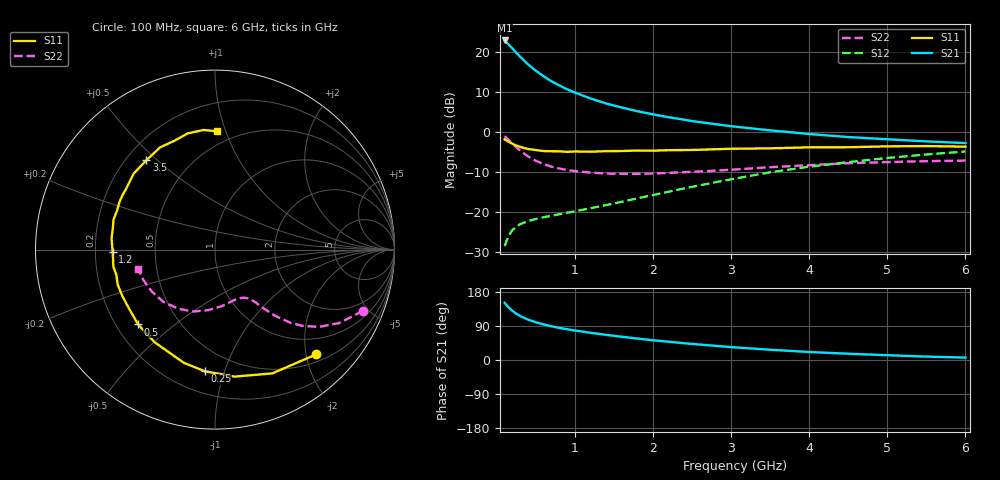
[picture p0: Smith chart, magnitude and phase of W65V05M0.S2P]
! SIEMENS Small Signal Semiconductors
! BFR193W
! Si NPN RF Bipolar Junction Transistor in SOT323
! VCE = 5 V  IC = 5 mA
! Common Emitter S-Parameters:  September  1992
# GHz  S  MA  R  50
!  f  S11  S21  S12  S22
! GHz  MAG  ANG  MAG  ANG  MAG  ANG  MAG  ANG
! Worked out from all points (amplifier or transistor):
!   28 points, 100 MHz to 6 GHz, reference 50 ohm
!   highest |S21| = 22.9 dB at 100 MHz (marker M1)
!   |S21| within 3 dB of that: start of sweep to 246.8 MHz
!   unconditionally stable (mu >= 1): 1.199 GHz to 2.565 GHz
!   at 300 MHz: K = 0.36, MSG = 20.9 dB, |S12| = -23.0 dB
!   at 1.5 GHz: K = 1.06, MAG = 10.7 dB, |S12| = -17.8 dB
!   at 6 GHz: K = 0.90, MSG = 1.0 dB, |S12| = -4.8 dB
!   lowest NFmin = 1.20 dB at 450 MHz
!   S11 on the Smith chart (normalised r, x): 100 MHz: 0.64, -2.19; 250 MHz: 0.34, -0.86; 500 MHz: 0.29, -0.38; 1.2 GHz: 0.27, -0.01; 3.5 GHz: 0.28, +0.46; 6 GHz: 0.40, +0.94
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0.1  0.811 -46.1  13.92 150.8  0.0378 67.1  0.8923 -22.5
0.15  0.76 -65.2  12.46 139.1  0.0508 58.7  0.8041 -30.6
0.2  0.7159 -81.3  11.05 129.7  0.0598 52.8  0.7211 -36.7
0.25  0.6798 -94.9  9.776 122.2  0.0665 48.3  0.6459 -41.1
0.3  0.6541 -105.4  8.685 116.1  0.0712 45.5  0.5884 -44.0
0.4  0.6161 -123.1  7.005 106.5  0.0777 42.3  0.4979 -47.8
0.5  0.5977 -135.8  5.828 99.6  0.0826 41.2  0.4392 -49.8
0.6  0.5806 -145.7  4.973 93.9  0.0869 41.6  0.3984 -51.5
0.7  0.5775 -153.5  4.31 89.0  0.0906 42.5  0.3712 -52.4
0.8  0.5761 -160.2  3.824 84.8  0.0945 43.8  0.3519 -53.7
0.9  0.5674 -165.6  3.424 81.2  0.0986 45.4  0.3372 -54.6
1  0.5741 -170.4  3.118 77.8  0.103 47.3  0.3276 -56.0
1.2  0.57 -178.7  2.628 71.8  0.1125 50.3  0.3122 -59.0
1.4  0.5789 174.4  2.279 66.3  0.1231 53.5  0.3048 -62.3
1.6  0.5812 168.5  2.028 61.3  0.1354 56.3  0.3013 -66.0
1.8  0.5896 163.5  1.824 56.6  0.1492 58.7  0.3013 -70.2
2.2  0.5948 153.5  1.534 48.2  0.1805 61.9  0.3097 -78.5
3  0.6203 136.8  1.185 34.0  0.2583 62.7  0.3396 -96.5
3.5  0.6275 127.6  1.052 27.1  0.3153 60.3  0.3655 -109.3
4.5  0.6477 110.1  0.868 16.6  0.4226 51.9  0.4091 -134.4
5.5  0.6697 95.5  0.766 9.0  0.5263 42.1  0.4345 -157.4
6  0.6589 88.9  0.73 6.4  0.5733 36.4  0.4416 -166.2
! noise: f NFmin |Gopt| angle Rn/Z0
0.45  1.2  0.26  102  0.14
0.9  1.25  0.38  145  0.12
1.8  2.05  0.56  -161  0.12
